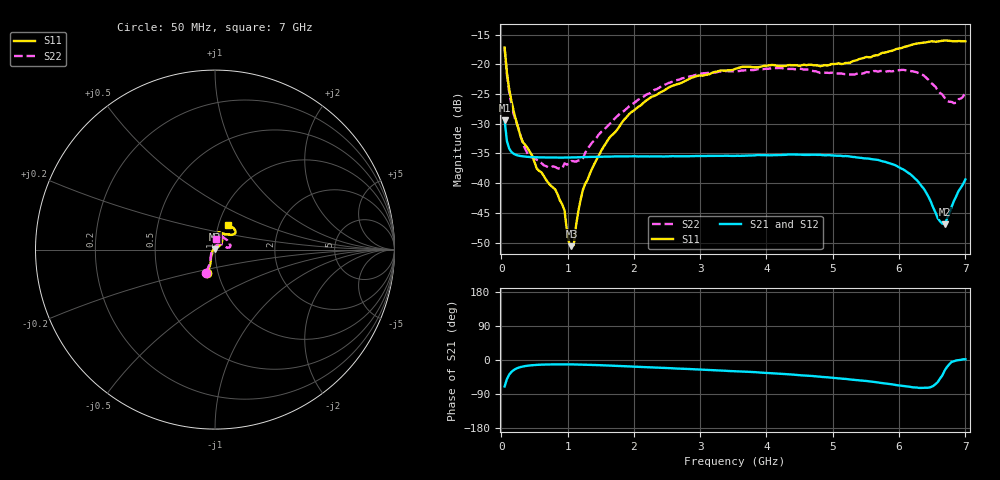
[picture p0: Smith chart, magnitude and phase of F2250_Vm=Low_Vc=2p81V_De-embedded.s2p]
! Integrated Device Technology
! Corporate Headquarters
! 6024 Silver Creek Valley Road
! San Jose, CA 95138  USA
! Phone:  1-408-284-8200
! Toll Free:  1-800-223-1366
! Webpage:  http://www.idt.com/
! Timing and RF Division
! 515 Groton Road, Suite 102
! Westford, MA 01886-6024
! Device:  F2250
! Description: Voltage Variable RF Attenuator
! Frequency:  50.0 -  6000.00 MHz
! Package:  3x3 mm Thin QFN Plastic Package: 16 pin
! Ports:  2 RF, 3 DC
!  Pin  1  = GND
!  Pin  2  = NC
!  Pin  3  = RF1  = Port 1
!  Pin  4  = NC
!  Pin  5  = GND
!  Pin  6  = GND
!  Pin  7  = GND
!  Pin  8  = GND
!  Pin  9  = NC
!  Pin 10  = RF2  = Port 2
!  Pin 11  = NC
!  Pin 12  = GND
!  Pin 13  = GND
!  Pin 14  = VCNTRL
!  Pin 15  = VDD
!  Pin 16  = VMODE
! Vcntrl:  2.810 Volts
! Vmode:  +0.000 Volts
! Vdd:  +3.30  Volts
! Current:  1.175 mA
! Data:  The device was measured on a the F2250 evaluation board which has
!  individual transmission lines to the RF pins.  Data was collected
!  using a calibrated network analyzer.  The evaluation board was
!  de-embedded using a TRL calibration technique.
!  The reference plane is the edge of the package pin.
! Misc:  SN 10
!  Action Tracker AT0258
! Date Measured:  2014-11-26
! Date:  2015-10-15  MJV
! Note:
!  Integrated Device Technology supplies this data as a sample of measured
!  data at the package pin for this product.  Your particular data for this
!  product may vary.
!  Data was taken at 25 degrees C.
!  Integrated Device Technology reserves the right to change this data at anytime.
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# GHz S dB R 50
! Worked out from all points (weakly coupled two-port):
!   201 points, 50 MHz to 7 GHz, reference 50 ohm
!   highest |S21| = -29.41 dB at 50 MHz (marker M1); lowest = -46.9 dB at 6.687 GHz (marker M2)
!   lowest |S11| = -50.6 dB at 1.058 GHz (marker M3), VSWR 1.01, Z = 49.8 + j0.247 ohm
!   |S11| at or under -10 dB: start of sweep to end of sweep
!   |S22| runs from -37.5 to -17.3 dB; largest |S21 - S12| = 5.6e-05
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0.05  -17.18 -108.6  -29.41 -69.8  -29.41 -69.8  -17.28 -111.0
0.08475  -21.45 -107.5  -32.92 -50.3  -32.91 -50.4  -21.74 -110.2
0.15425  -26.23 -116.6  -34.76 -31.1  -34.76 -31.1  -26.81 -122.5
0.29325  -32.21 -127.9  -35.43 -18.5  -35.43 -18.5  -32.10 -137.3
0.3975  -34.10 -141.8  -35.56 -15.0  -35.56 -15.0  -35.04 -160.4
0.91875  -43.53 157.8  -35.69 -11.5  -35.69 -11.5  -37.53 133.6
0.9535  -44.60 169.8  -35.68 -11.5  -35.68 -11.5  -36.66 131.1
1.023  -50.01 143.6  -35.67 -11.6  -35.68 -11.6  -36.64 115.9
1.05775  -50.58 123.0  -35.67 -11.6  -35.67 -11.6  -36.27 110.7
1.0925  -50.41 89.9  -35.66 -11.7  -35.65 -11.7  -36.31 106.3
1.162  -44.67 57.1  -35.64 -11.9  -35.64 -11.9  -36.18 95.5
1.2315  -41.09 44.3  -35.61 -12.1  -35.61 -12.1  -35.80 85.8
1.6485  -32.11 41.9  -35.52 -14.6  -35.52 -14.6  -29.88 64.6
1.96125  -28.04 42.2  -35.46 -17.2  -35.46 -17.2  -26.81 56.8
2.37825  -24.87 47.3  -35.48 -20.3  -35.48 -20.3  -23.98 56.8
3.525  -20.79 72.5  -35.40 -29.5  -35.40 -29.5  -21.19 74.7
4.7065  -20.17 72.4  -35.20 -42.6  -35.20 -42.6  -21.14 72.2
5.85325  -17.81 40.5  -36.64 -63.3  -36.63 -63.4  -21.14 23.0
6.27025  -16.51 40.0  -39.51 -72.8  -39.51 -72.7  -21.36 9.7
6.68725  -15.99 48.7  -46.87 -27.8  -46.86 -27.4  -25.64 28.6
6.861  -16.13 55.1  -42.20 -1.3  -42.16 -1.3  -26.46 57.9
7  -16.13 63.2  -39.36 1.9  -39.32 1.8  -24.63 83.1
